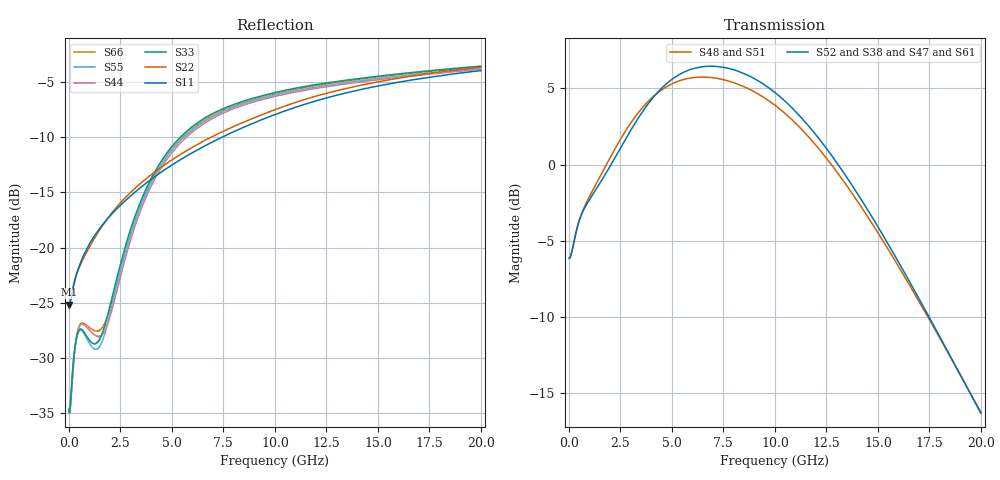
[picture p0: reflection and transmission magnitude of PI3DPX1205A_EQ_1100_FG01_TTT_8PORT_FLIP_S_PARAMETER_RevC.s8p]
! NPort=8 DATA=2000 NOISE=0 GROUPDELAY=0 COMPLEX_DATAFORMAT=POLAR
! NumOfBlock=1 NumOfParam=0
! .MODEL Smodel S TSTONEFILE=PI3DPX1205A_EQ_1100_FG01_TTT_8PORT_FLIP_S_PARAMETER_RevC.s8p TYPE=S
!  -- The above .MODEL line can be used for the S element in the netlist.
! The s parameter is extracted from the linear redriver, it is not bi-directional;
! only s(5,1)s(6,2)s(3,7)s(4,8) should be the insertion loss
!  Port definition:
!  Port1 = AIP
!  Port2 = AIN
!  Port3 = BOP
!  Port4 = BON
!  Port5 = AOP
!  Port6 = AON
!  Port7 = BIP
!  Port8 = BIN
# Hz S MA R  50
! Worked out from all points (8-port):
!   2000 points, 10 MHz to 20 GHz, reference 50 ohm
!   strongest paths, dB at 10 MHz, 5.01 GHz, 10.01 GHz, 15.01 GHz, 20 GHz:
!     S52: -6.1, 5.6, 4.7, -4.1, -16.3
!     S38: -6.1, 5.6, 4.7, -4.1, -16.3
!     S47: -6.1, 5.6, 4.7, -4.0, -16.2
!     S61: -6.1, 5.6, 4.7, -4.1, -16.2
!     S48: -6.1, 5.3, 3.9, -4.5, -16.2
!     S51: -6.1, 5.3, 3.9, -4.5, -16.2
!   lowest |S11| = -25.2 dB at 10 MHz (marker M1), VSWR 1.12, Z = 44.8 - j0.115 ohm
!   |S11| at or under -10 dB: start of sweep to 7.452 GHz
